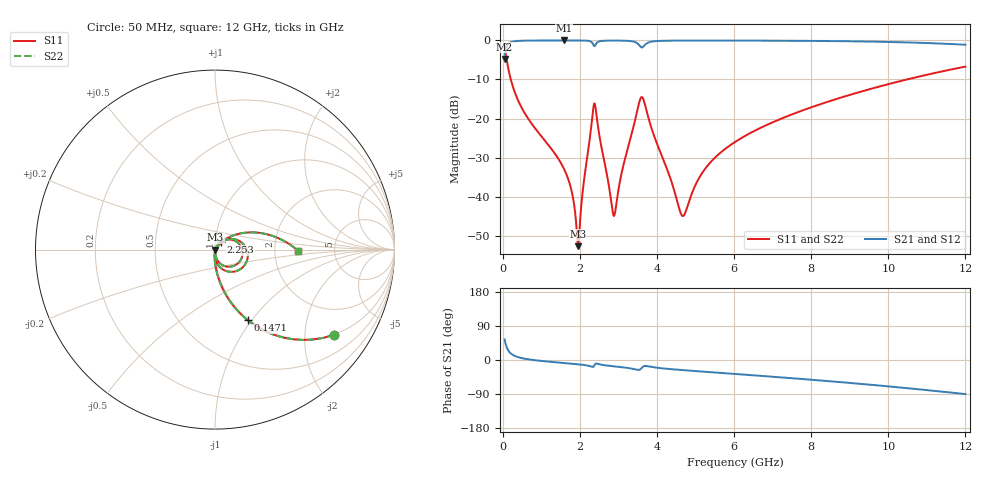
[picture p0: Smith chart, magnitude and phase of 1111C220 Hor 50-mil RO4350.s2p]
# GHz S MA R 50
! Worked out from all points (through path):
!   1601 points, 50 MHz to 12 GHz, reference 50 ohm
!   highest |S21| = -0.01 dB at 1.589 GHz (marker M1); lowest = -4.8 dB at 50 MHz (marker M2)
!   group delay of S21, straight-line fit = 21.8 ps
!   lowest |S11| = -52.7 dB at 1.955 GHz (marker M3), VSWR 1.00, Z = 50.2 - j0.0916 ohm
!   |S11| at or under -10 dB: 211 MHz to 10.48 GHz (10.27 GHz wide, 192 % of centre)
!   |S22| runs from -52.7 to -1.8 dB; largest |S21 - S12| = 0
!   S11 on the Smith chart (normalised r, x): 50 MHz: 0.99, -2.81; 147.1 MHz: 0.99, -0.95; 2.253 GHz: 1.06, +0.09; 12 GHz: 2.72, -0.04
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0.05  0.8167 -35.5  0.5768 54.5  0.5768 54.5  0.8167 -35.5
0.1470937  0.4326 -65.2  0.9012 24.8  0.9012 24.8  0.4326 -65.2
0.2665938  0.2542 -76.7  0.9667 13.2  0.9667 13.2  0.2542 -76.7
0.5205313  0.1295 -85.3  0.9909 4.4  0.9909 4.4  0.1295 -85.3
1.588563  0.02277 -95.0  0.9985 -7.9  0.9985 -7.9  0.02277 -95.0
1.78275  0.0121 -92.6  0.9983 -9.7  0.9983 -9.7  0.0121 -92.6
1.954531  0.002324 -23.1  0.9976 -11.3  0.9976 -11.3  0.002324 -23.1
2.044156  0.008294 54.5  0.9966 -12.3  0.9966 -12.3  0.008294 54.5
2.253281  0.05271 52.8  0.9795 -15.9  0.9795 -15.9  0.05271 52.8
2.342906  0.1276 20.3  0.8967 -18.1  0.8967 -18.1  0.1276 20.3
2.402656  0.1434 -36.9  0.8697 -10.2  0.8697 -10.2  0.1434 -36.9
2.888125  0.005675 -13.9  0.9942 -16.7  0.9942 -16.7  0.005675 -13.9
3.134594  0.02567 51.9  0.9913 -19.5  0.9913 -19.5  0.02567 51.9
3.582719  0.1841 -7.5  0.8215 -23.5  0.8215 -23.5  0.1841 -7.5
3.69475  0.1478 -56.6  0.8834 -15.7  0.8834 -15.7  0.1478 -56.6
4.038312  0.04282 -89.9  0.9837 -20.9  0.9837 -20.9  0.04282 -89.9
4.673156  0.005638 -20.7  0.9941 -26.7  0.9941 -26.7  0.005638 -20.7
5.225844  0.0219 47.7  0.9952 -30.9  0.9952 -30.9  0.0219 47.7
6.025  0.05008 48.8  0.9946 -36.8  0.9946 -36.8  0.05008 48.8
8.019156  0.1401 36.2  0.9857 -52.2  0.9857 -52.2  0.1401 36.2
10.01331  0.2765 19.3  0.9556 -69.7  0.9556 -69.7  0.2765 19.3
12  0.4618 -0.7  0.8803 -89.9  0.8803 -89.9  0.4618 -0.7
